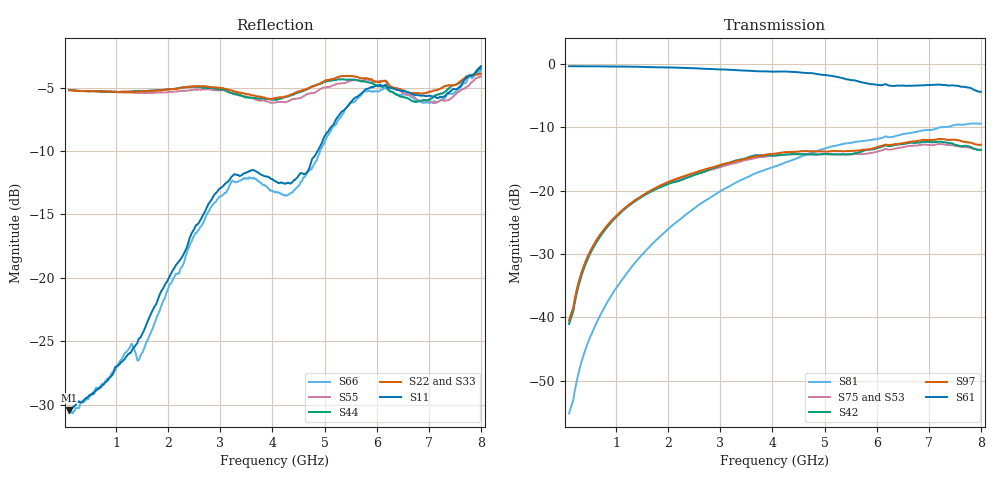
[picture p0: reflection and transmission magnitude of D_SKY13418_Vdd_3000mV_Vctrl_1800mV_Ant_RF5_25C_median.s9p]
# GHz S DB R 50
! THRU S21 mag phase subtraction.
! HALF_THRU
! EN33-165-011-v1_HALF_THRU_1 EN33-165-011-v1_HALF_THRU_2 EN33-165-011-v1_HALF_THRU_3 EN33-165-011-v1_HALF_THRU_4 EN33-165-011-v1_HALF_THRU_5 EN33-165-011-v1_HALF_THRU_6 EN33-165-011-v1_HALF_THRU_7 EN33-165-011-v1_HALF_THRU_8 EN33-165-011-v1_HALF_THRU_9
! THRU Ports: 1 2
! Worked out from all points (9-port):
!   801 points, 100 MHz to 8 GHz, reference 50 ohm
!   strongest paths, dB at 100 MHz, 2.075 GHz, 4.05 GHz, 6.025 GHz, 8 GHz:
!     S61: -0.4, -0.6, -1.2, -3.3, -4.4
!     S97: -40.5, -18.4, -14.2, -13.1, -12.8
!     S42: -41.0, -18.8, -14.5, -13.3, -13.6
!     S75: -40.6, -18.6, -14.5, -13.8, -13.5
!     S53: -41.0, -18.8, -14.6, -13.8, -13.6
!     S81: -55.1, -25.5, -16.2, -11.8, -9.4
!   lowest |S11| = -30.4 dB at 100 MHz (marker M1), VSWR 1.06, Z = 53.1 + j0.0888 ohm
!   |S11| at or under -10 dB: start of sweep to 4.871 GHz
